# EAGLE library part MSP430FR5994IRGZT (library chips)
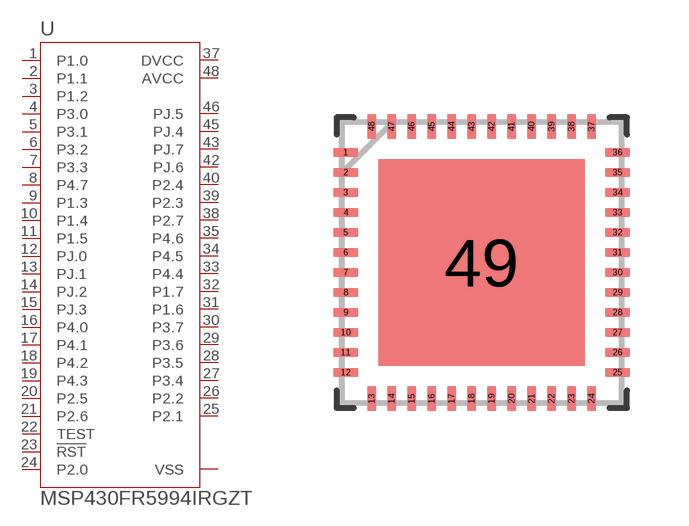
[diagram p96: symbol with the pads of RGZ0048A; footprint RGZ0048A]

Designator prefix U

## MSP430FR5994IRGZT (MANUFACTURER_PART_NUMBER: MSP430FR5994IRGZT; VENDOR: Texas Instruments)  [RGZ0048A]
1  P1.0
2  P1.1
3  P1.2
4  P3.0
5  P3.1
6  P3.2
7  P3.3
8  P4.7
9  P1.3
10  P1.4
11  P1.5
12  PJ.0
13  PJ.1
14  PJ.2
15  PJ.3
16  P4.0
17  P4.1
18  P4.2
19  P4.3
20  P2.5
21  P2.6
22  TEST  in
23  !RST
24  P2.0
25  P2.1
26  P2.2
27  P3.4
28  P3.5
29  P3.6
30  P3.7
31  P1.6
32  P1.7
33  P4.4
34  P4.5
35  P4.6
37  DVCC  pwr
38  P2.7
39  P2.3
40  P2.4
42  PJ.6
43  PJ.7
45  PJ.4
46  PJ.5
48  AVCC  pwr

## Footprint RGZ0048A (pad centres in mm)
smd 0.61 x 0.229: 1 -3.4,2.75; 2 -3.4,2.25; 3 -3.4,1.75; 4 -3.4,1.25; 5 -3.4,0.75; 6 -3.4,0.25; 7 -3.4,-0.25; 8 -3.4,-0.75; 9 -3.4,-1.25; 10 -3.4,-1.75; 11 -3.4,-2.25; 12 -3.4,-2.75; 25 3.4,-2.75; 26 3.4,-2.25; 27 3.4,-1.75; 28 3.4,-1.25; 29 3.4,-0.75; 30 3.4,-0.25; 31 3.4,0.25; 32 3.4,0.75; 33 3.4,1.25; 34 3.4,1.75; 35 3.4,2.25; 36 3.4,2.75
smd 0.229 x 0.61: 13 -2.75,-3.4; 14 -2.25,-3.4; 15 -1.75,-3.4; 16 -1.25,-3.4; 17 -0.75,-3.4; 18 -0.25,-3.4; 19 0.25,-3.4; 20 0.75,-3.4; 21 1.25,-3.4; 22 1.75,-3.4; 23 2.25,-3.4; 24 2.75,-3.4; 37 2.75,3.4; 38 2.25,3.4; 39 1.75,3.4; 40 1.25,3.4; 41 0.75,3.4; 42 0.25,3.4; 43 -0.25,3.4; 44 -0.75,3.4; 45 -1.25,3.4; 46 -1.75,3.4; 47 -2.25,3.4; 48 -2.75,3.4
smd 5.156 x 5.156: 49 0,0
